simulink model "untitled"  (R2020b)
settings: Solver=VariableStepAuto  StartTime=0.0  StopTime=10.0  RelTol=1e-3
undefined symbols (not defined in the file or in its folder): bm, Jm, Kb, Kt, La, Ra
libraries: fl_lib x4, nesl_utility x3, ee_lib x1

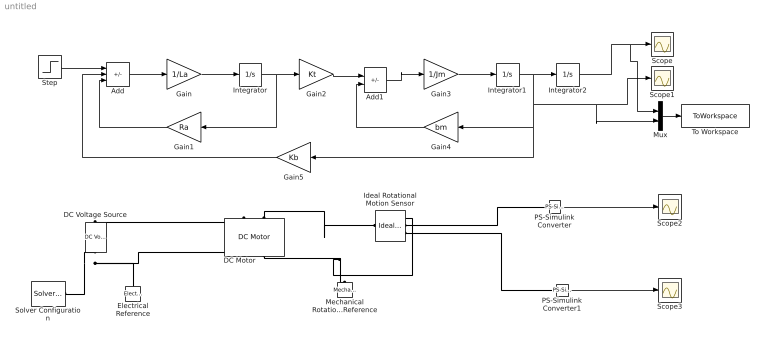
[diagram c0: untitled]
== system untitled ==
  Add : Sum  Inputs=+--
  Add1 : Sum  Inputs=+-
  DC Motor : ee_lib/Electromechanical/Brushed Motors/DC Motor  field_option=ee.enum.field_option.pm  Rf=100 Ohm  Lf=1 H  Laf=0.15 H  If0=0 A  parameterization=ee.enum.dcparam_option.circuit_param  Ra=Ra Ohm  La=La H  emf_or_torque=ee.enum.emf_or_torque.ki  Kv=Kt V/rpm  Ki=Kt N*m/A  T_stall=0.24e-3 N*m  w_max=19100 rpm  w_rated=15000 rpm  P_rated=0.08 W  V_rated=1.5 V  J=Jm kg*m^2  lam_param=ee.enum.lam_param.damping  lam=bm N*m/(rad/s)  i_noload=0 A  V_i_noload=1.5 V  speed0=0 rpm  enable_fault_armature=ee.enum.faults.faultEnable.no  rev_faulted=1 / 3  G_faulted_armature=1e-5 S  fault_trigger_armature=ee.enum.faults.faultTrigger.temporal  t_fault_armature=1 s  max_permissible_current_armature=inf A  t_fail_on_current_armature=1 s  enable_fault_field=ee.enum.faults.faultEnable.no  G_faulted_field=1e-5 S  fault_trigger_field=ee.enum.faults.faultTrigger.temporal  t_fault_field=1 s  max_permissible_current_field=inf A  t_fail_on_current_field=1 s  fault_action=ee.enum.faults.faultAction.none  alpha=3.93e-3 1/K  Tmeas=25 degC  thermal_mass=100 J/K  initial_temperature=25 degC
  DC Voltage Source : fl_lib/Electrical/Electrical Sources/DC Voltage Source  v0=1 V
  Electrical Reference : fl_lib/Electrical/Electrical Elements/Electrical Reference
  Gain : Gain  Gain=1/La
  Gain1 : Gain  Gain=Ra
  Gain2 : Gain  Gain=Kt
  Gain3 : Gain  Gain=1/Jm
  Gain4 : Gain  Gain=bm
  Gain5 : Gain  Gain=Kb
  Ideal Rotational Motion Sensor : fl_lib/Mechanical/Mechanical Sensors/Ideal Rotational Motion Sensor  wrap_angle=simscape.enum.onoff.off  offset=0 rad
  Integrator : Integrator
  Integrator1 : Integrator
  Integrator2 : Integrator
  Mechanical Rotational Reference : fl_lib/Mechanical/Rotational Elements/Mechanical Rotational Reference
  Mux : Mux  Inputs=2
  PS-Simulink Converter : nesl_utility/PS-Simulink Converter  PhysicalDomain=network_engine_domain  SubClassName=ps_output  LeftPortType=input  RightPortType=output  PseudoPeriodic=off  Frequencies=[]  Unit=inherit  AffineConversion=off
  PS-Simulink Converter1 : nesl_utility/PS-Simulink Converter  PhysicalDomain=network_engine_domain  SubClassName=ps_output  LeftPortType=input  RightPortType=output  PseudoPeriodic=off  Frequencies=[]  Unit=inherit  AffineConversion=off
  Scope{,1..3} (4 alike) : Scope
  Solver Configuration : nesl_utility/Solver Configuration  PhysicalDomain=network_engine_domain  SubClassName=solver  LeftPortType=input  RightPortType=generic  Tones=[]  Harmonics=[]  SimulateNoise=off  Profile=off  UseLocalSampling=off  EnableSwitchedLinearOptims=on  FrequencyDomain=off  UseCCode=off  RelTol=0.001  AbsTol=1e-06  MinStep=1e-09  ToWorkspace=off  RevertToSquareIcSolve=off  NumHomotopyIterations=100  PhasorMode=off  PhasorModeNumHarmonics=1  DoDC=off  ResidualTolerance=1e-09  UseLocalSolver=off  LocalSolverChoice=NE_BACKWARD_EULER_ADVANCER  LocalSolverSampleTime=0.001  DoFixedCost=off  MaxNonlinIter=3  MaxModeIter=2  ComputeImpulses=off  ImpulseIterations=2  LinearAlgebra=auto  EquationFormulation=NE_TIME_EF  DelaysMemoryBudget=1024  AutomaticFiltering=on  FilteringTimeConstant=0.001  PartitionStorageMethod=AS_NEEDED  PartitionMemoryBudget=1024  PartitionMethod=ROBUST
  Step : Step  Time=0  SampleTime=0
  To Workspace : ToWorkspace  VariableName=simout  SaveFormat=Timeseries  SampleTime=-1
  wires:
  Gain/1 -> Integrator/1
  Add/1 -> Gain/1
  Gain1/1 -> Add/3
  Integrator/1 -> Gain2/1, Gain1/1
  Gain3/1 -> Integrator1/1
  Integrator1/1 -> Integrator2/1, Gain5/1, Gain4/1, Mux/2, Scope1/1
  Add1/1 -> Gain3/1
  Gain2/1 -> Add1/1
  Gain4/1 -> Add1/2
  Step/1 -> Add/1
  Gain5/1 -> Add/2
  Integrator2/1 -> Mux/1, Scope/1
  Mux/1 -> To Workspace/1
  PS-Simulink Converter/1 -> Scope2/1
  PS-Simulink Converter1/1 -> Scope3/1
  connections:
  DC Motor/LConn1 -- DC Voltage Source/LConn1
  Solver Configuration/RConn1 -- Electrical Reference/LConn1 -- DC Motor/RConn1 -- DC Voltage Source/RConn1
  DC Motor/RConn2 -- Ideal Rotational Motion Sensor/RConn1 -- Mechanical Rotational Reference/LConn1
  DC Motor/LConn2 -- Ideal Rotational Motion Sensor/LConn1
  PS-Simulink Converter/LConn1 -- Ideal Rotational Motion Sensor/RConn2
  PS-Simulink Converter1/LConn1 -- Ideal Rotational Motion Sensor/RConn3
